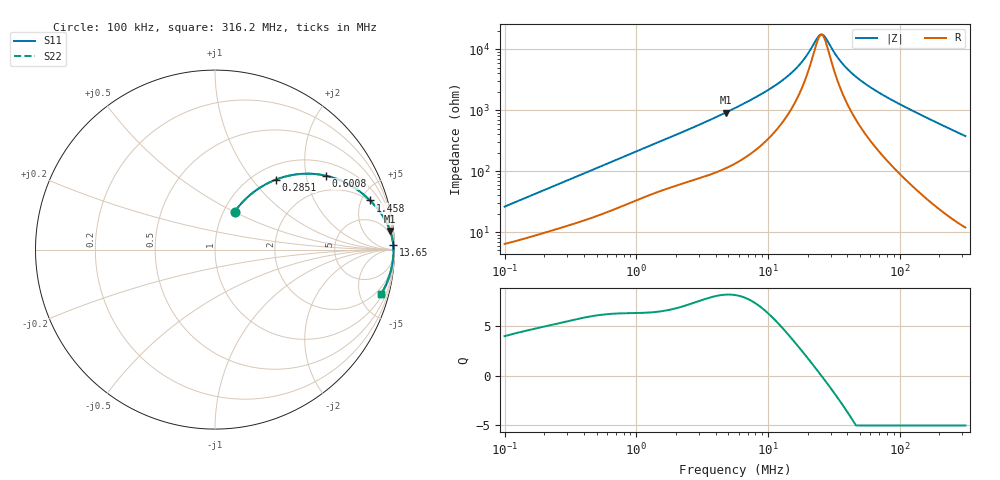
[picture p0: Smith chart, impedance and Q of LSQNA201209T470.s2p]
! LSQNA201209T470  S-PARAMETER MODEL  ( General Type )
! Model Generated by TAIYO YUDEN Corporation (http://www.ty-top.com)
! Version 2.0
! TAIYO YUDEN Control No. 100810NF25SB-FAC
! Copyright(c) 2007 TAIYO YUDEN CO.,LTD. All Rights Reserved.
! Product Description (link to TY-COMPAS)
! https://ds.yuden.co.jp/TYCOMPAS/or/detail?pn=LSQNA201209T470M&u=M
! Products Name : Inductors
! Characteristics :
!  Inductance : 47 uH , SRF(min) : 11 MHz , DC Resistance(max) : 5.46 Ohm
!  Rated Current : Saturation :100 mA , Temp Rise : 140 mA (40 degC)
!  Case Size : 2.0 x 1.25 / 0.079 x 0.049 [mm/inch] , Thickness : 0.9 / 0.035 [mm/inch]
!  (Conditions: Temperature = 25 degC , DC Bias Current/Voltage = 0A / 0V)
! External Node Assignments :
!  1  o---GGG---o  2
! GND o---------o GND
! Frequency Range : 0.1MHz  -  316.199832MHz  [ 402 STEP ]
# MHz S RI R 50
! Freq[MHz].  S11 Real  S11 Imag  S21 Real  S21 Imag  S12 Real  S12 Imag  S22 Real  S22 Imag
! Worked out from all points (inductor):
!   401 points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, 100 kHz to 316.2 MHz, reference 50 ohm
!   read as one part in series: L = 39.6 uH near 104.1 kHz
!   highest Q = 8.15 at 4.786 MHz (marker M1), where L = 30.2 uH
!   self-resonance near 24.97 MHz
!   S11 on the Smith chart (normalised r, x): 100 kHz: 1.13, +0.51; 285.1 kHz: 1.24, +1.32; 600.8 kHz: 1.42, +2.62; 1.458 MHz: 1.91, +5.85; 13.65 MHz: 16, +66; 316.2 MHz: 1.24, -7.50
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0.1  0.1106 0.2121  0.8894 -0.2121  0.8894 -0.2121  0.1106 0.2121
0.172285  0.1995 0.3079  0.8005 -0.3079  0.8005 -0.3079  0.1995 0.3079
0.285099  0.3387 0.3898  0.6613 -0.3898  0.6613 -0.3898  0.3387 0.3898
0.385695  0.448 0.4184  0.552 -0.4184  0.552 -0.4184  0.448 0.4184
0.600816  0.6196 0.4113  0.3804 -0.4113  0.3804 -0.4113  0.6196 0.4113
0.935921  0.7646 0.3521  0.2354 -0.3521  0.2354 -0.3521  0.7646 0.3521
1.457932  0.8636 0.2741  0.1364 -0.2741  0.1364 -0.2741  0.8636 0.2741
1.487603  0.8671 0.2706  0.1329 -0.2706  0.1329 -0.2706  0.8671 0.2706
4.786098  0.9757 0.1045  0.0243 -0.1045  0.0243 -0.1045  0.9757 0.1045
5.623165  0.9808 0.0888  0.0192 -0.0888  0.0192 -0.0888  0.9808 0.0888
9.494636  0.9901 0.0487  0.00991 -0.0487  0.00991 -0.0487  0.9901 0.0487
13.6451  0.9928 0.0283  0.00723 -0.0283  0.00723 -0.0283  0.9928 0.0283
17.73068  0.9937 0.0158  0.00625 -0.0158  0.00625 -0.0158  0.9937 0.0158
21.68824  0.9942 0.00689  0.00585 -0.00689  0.00585 -0.00689  0.9942 0.00689
24.47506  0.9943 0.0017  0.00572 -0.0017  0.00572 -0.0017  0.9943 0.0017
26.52916  0.9943 -0.00174  0.00567 0.00174  0.00567 0.00174  0.9943 -0.00174
34.47245  0.9943 -0.0131  0.00574 0.0131  0.00574 0.0131  0.9943 -0.0131
42.16686  0.994 -0.0224  0.00604 0.0224  0.00604 0.0224  0.994 -0.0224
55.90748  0.9931 -0.0371  0.00691 0.0371  0.00691 0.0371  0.9931 -0.0371
83.65039  0.9903 -0.0634  0.00966 0.0634  0.00966 0.0634  0.9903 -0.0634
165.9452  0.9756 -0.1332  0.0244 0.1332  0.0244 0.1332  0.9756 -0.1332
316.1998  0.927 -0.2448  0.073 0.2448  0.073 0.2448  0.927 -0.2448
